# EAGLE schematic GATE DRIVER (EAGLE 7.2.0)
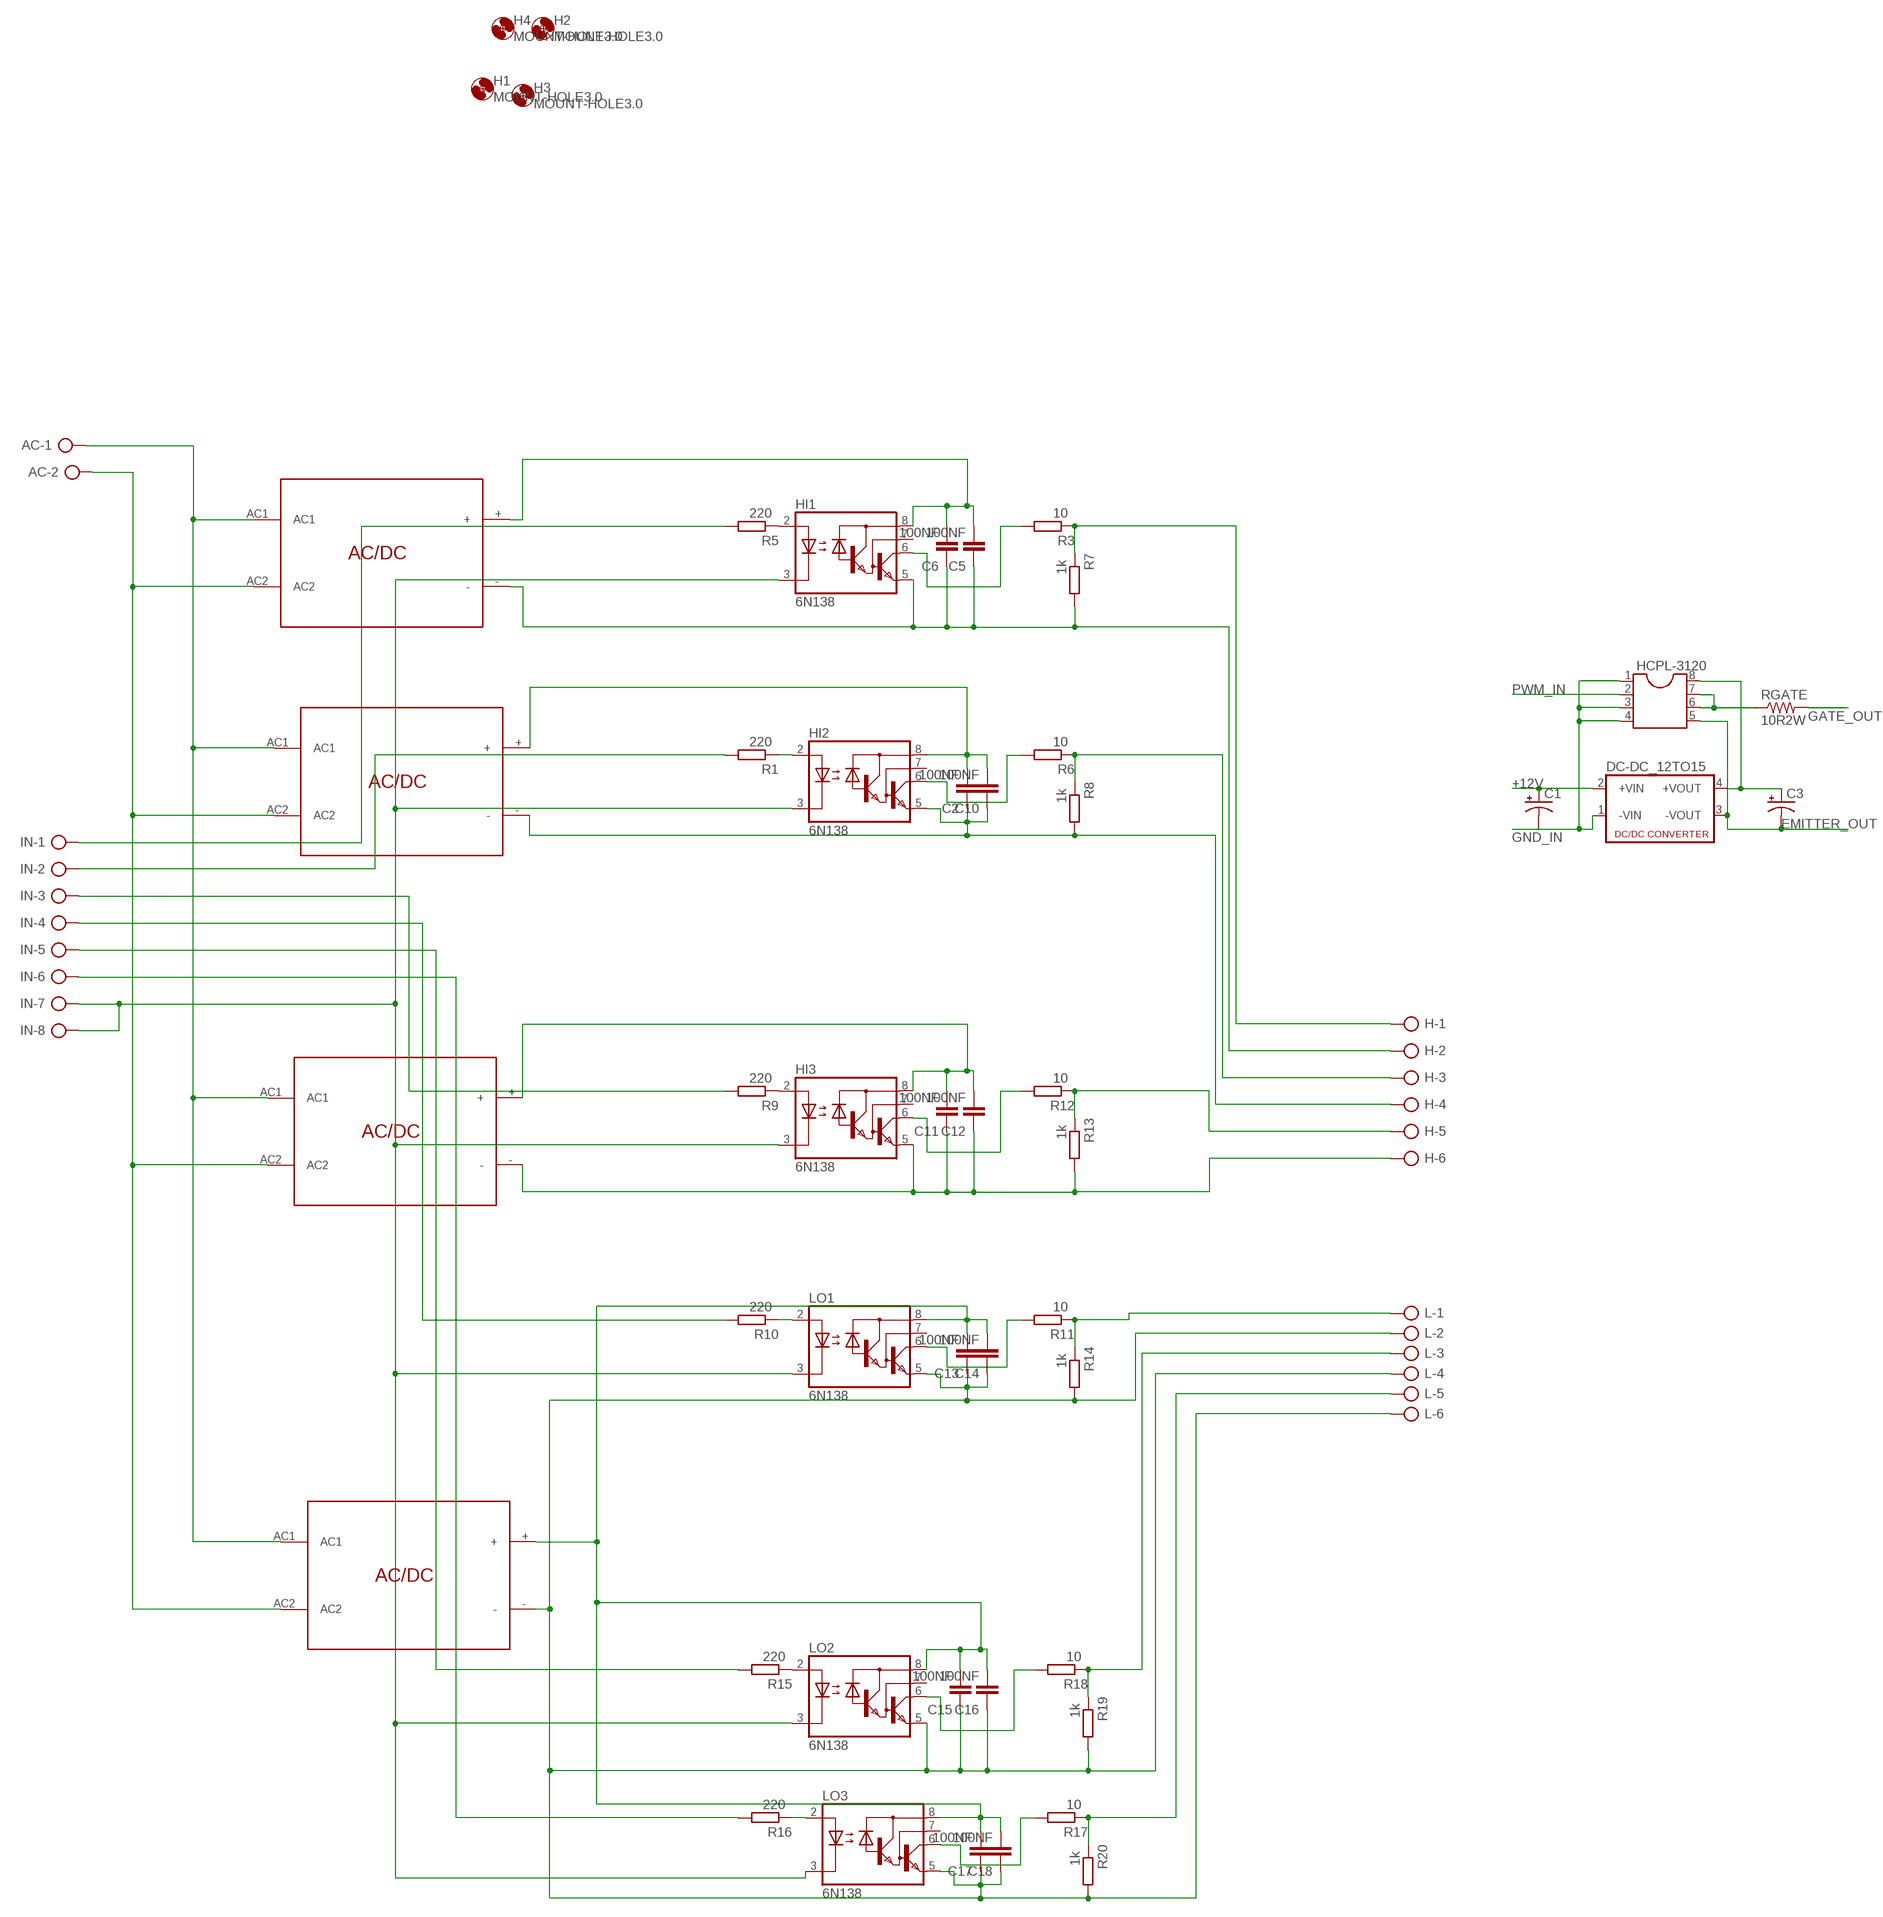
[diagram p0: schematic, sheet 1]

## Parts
AC  AK300/2  [AK300/2]
C1  CPOL-US085CS-1W  [085CS_1W]
C2  100NF  C0805  [R0805]
C3  CPOL-US085CS-1W  [085CS_1W]
C5  100NF  C0805  [R0805]
C6  100NF  C0805  [R0805]
C10  100NF  C0805  [R0805]
C11  100NF  C0805  [R0805]
C12  100NF  C0805  [R0805]
C13  100NF  C0805  [R0805]
C14  100NF  C0805  [R0805]
C15  100NF  C0805  [R0805]
C16  100NF  C0805  [R0805]
C17  100NF  C0805  [R0805]
C18  100NF  C0805  [R0805]
DC-DC_12TO15  NME  [NME]
H  AK300/6  [AK300/6]
H1  MOUNT-HOLE3.0  [3,0]
H2  MOUNT-HOLE3.0  [3,0]
H3  MOUNT-HOLE3.0  [3,0]
H4  MOUNT-HOLE3.0  [3,0]
HCPL-3120  DIL8  [DIL08]
HI1  6N138  [DIL08]
HI2  6N138  [DIL08]
HI3  6N138  [DIL08]
IN  AK300/8  [AK300/8]
L  AK300/6  [AK300/6]
LO1  6N138  [DIL08]
LO2  6N138  [DIL08]
LO3  6N138  [DIL08]
R1  220  R0805  [R0805]
R3  10  R0805  [R0805]
R5  220  R0805  [R0805]
R6  10  R0805  [R0805]
R7  1k  R0805  [R0805]
R8  1k  R0805  [R0805]
R9  220  R0805  [R0805]
R10  220  R0805  [R0805]
R11  10  R0805  [R0805]
R12  10  R0805  [R0805]
R13  1k  R0805  [R0805]
R14  1k  R0805  [R0805]
R15  220  R0805  [R0805]
R16  220  R0805  [R0805]
R17  10  R0805  [R0805]
R18  10  R0805  [R0805]
R19  1k  R0805  [R0805]
R20  1k  R0805  [R0805]
RGATE  10R2W  R-US_0204/5  [0204/5]
U$1  ADAPTOR  [ADAPTOR]
U$2  ADAPTOR  [ADAPTOR]
U$6  ADAPTOR  [ADAPTOR]
U$7  ADAPTOR  [ADAPTOR]

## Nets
+12V: C1.+ DC-DC_12TO15.2(+VIN)
EMITTER_OUT: C3.- DC-DC_12TO15.3(-VOUT) HCPL-3120.5
G2: HI1.3(C) HI2.3(C) HI3.3(C) IN.7 IN.8 LO1.3(C) LO2.3(C) LO3.3(C)
GATE_OUT: RGATE.2
GND_IN: DC-DC_12TO15.1(-VIN) HCPL-3120.1 HCPL-3120.3 HCPL-3120.4
HIGH1: H.5 R12.1 R13.1
HIGH2: L.3 R18.1 R19.1
LOW: H.3 R6.1 R8.1
LOW1: L.1 R11.1 R14.1
LOW2: L.5 R17.1 R20.1
N$1: IN.2 R1.2
N$2: H.1 R3.1 R7.1
N$3: HI2.2(A) R1.1
N$4: IN.1 R5.2
N$5: IN.3 R9.2
N$6: IN.4 R10.2
N$7: IN.5 R15.2
N$8: IN.6 R16.2
N$9: LO1.2(A) R10.1
N$10: LO1.6(VO) R11.2
N$11: HI1.6(VO) R3.2
N$12: HI3.6(VO) R12.2
N$14: AC.2 U$1.AC2 U$2.AC2 U$6.AC2 U$7.AC2
N$15: C2.2 C10.2 HI2.8(VCC) U$6.+
N$16: AC.1 U$1.AC1 U$2.AC1 U$6.AC1 U$7.AC1
N$17: C5.2 C6.2 HI1.8(VCC) U$7.+
N$20: HI1.2(A) R5.1
N$21: HCPL-3120.6 HCPL-3120.7 RGATE.1
N$23: C2.1 C10.1 H.4 HI2.5(GND) R8.2 U$6.-
N$24: C3.+ DC-DC_12TO15.4(+VOUT) HCPL-3120.8
N$25: HI2.6(VO) R6.2
N$27: C5.1 C6.1 H.2 HI1.5(GND) R7.2 U$7.-
N$28: C11.2 C12.2 HI3.8(VCC) U$2.+
N$40: C11.1 C12.1 H.6 HI3.5(GND) R13.2 U$2.-
N$41: HI3.2(A) R9.1
N$42: LO3.2(A) R16.1
N$43: LO3.6(VO) R17.2
N$44: LO2.6(VO) R18.2
N$46: C13.2 C14.2 C15.2 C16.2 C17.2 C18.2 LO1.8(VCC) LO2.8(VCC) LO3.8(VCC) U$1.+
N$50: C13.1 C14.1 C15.1 C16.1 C17.1 C18.1 L.2 L.4 L.6 LO1.5(GND) LO2.5(GND) LO3.5(GND) R14.2 R19.2 R20.2 U$1.-
N$51: LO2.2(A) R15.1
PWM_IN: HCPL-3120.2
Unconnected: C1.- HI1.7(VB) HI2.7(VB) HI3.7(VB) LO1.7(VB) LO2.7(VB) LO3.7(VB)

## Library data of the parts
AC = con-ptr500:AK300/2: CONNECTOR; OC_FARNELL: unknown; OC_NEWARK: unknown
C1 C3 = rcl:CPOL-US: POLARIZED CAPACITOR, American symbol
C2 C5 C6 C10-C18 = Charger:C0805
DC-DC_12TO15 = dc-dc-converter:NME: DC-DC CONVERTER; MF: C & D TECHNOLOGIES, INC; MPN: NME1205D; OC_FARNELL: 1021466; OC_NEWARK: 98B8198
H L = con-ptr500:AK300/6: CONNECTOR; OC_FARNELL: unknown; OC_NEWARK: unknown
H1-H4 = holes:MOUNT-HOLE: MOUNTING HOLE with drill center marker
HCPL-3120 = ic-package:DIL8: Dual In Line / Socket
HI1-HI3 LO1-LO3 = optocoupler:6N138: MOTOROLA OPTO COUPLER; MF: VISHAY/TELEFUNKEN; MPN: 6N138; OC_FARNELL: 9860150; OC_NEWARK: 35K5294
IN = con-ptr500:AK300/8: CONNECTOR; OC_FARNELL: unknown; OC_NEWARK: unknown
R1 R3 R5-R20 = Charger:R0805
RGATE = rcl:R-US_: RESISTOR, American symbol
U$1 U$2 U$6 U$7 = adaptor_rizani:ADAPTOR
